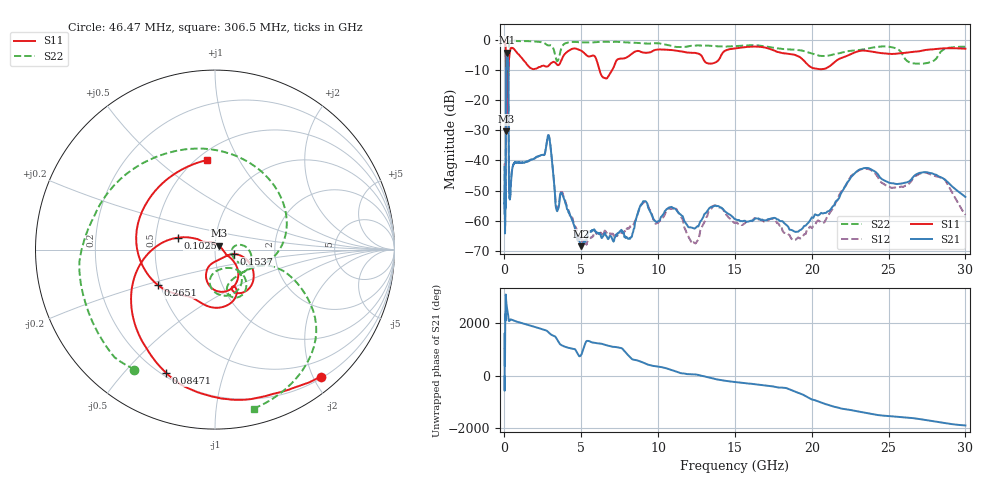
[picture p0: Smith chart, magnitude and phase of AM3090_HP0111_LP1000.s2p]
! Date/Time: Thu, Feb 28, 2019 2:01 PM
! Network Analyzer: Agilent Technologies E8364B Rev: A.07.50.67
! Sweep from 0.010 to 30.000 GHz, 1601 Points, Sweep Type: LOG
! Power Supply: 5.023 V, 0.002 A
# Hz S DB R 50
!freq MagS11 AngS11 MagS21 AngS21 MagS12 AngS12 MagS22 AngS22
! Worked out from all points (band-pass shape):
!   1601 points, 10 MHz to 30 GHz, reference 50 ohm
!   highest |S21| = -4.21 dB at 160.7 MHz (marker M1); lowest = -68.5 dB at 4.977 GHz (marker M2)
!   |S21| within 3 dB of the highest: 113.8 MHz to 240.5 MHz (126.7 MHz wide, 71.5 % of centre)
!   lowest |S11| = -30.3 dB at 110.4 MHz (marker M3), VSWR 1.06, Z = 52.1 + j2.32 ohm
!   |S11| at or under -10 dB: 100.6 MHz to 223.6 MHz (123 MHz wide, 75.9 % of centre); 234.8 MHz to 255.3 MHz (20.52 MHz wide, 8.37 % of centre); 6.184 GHz to 7.008 GHz (823.9 MHz wide, 12.5 % of centre)
!   |S22| runs from -20.7 to -0.1 dB; largest |S21 - S12| = 0.016
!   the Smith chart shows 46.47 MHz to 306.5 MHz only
!   S11 on the Smith chart (normalised r, x): 46.47 MHz: 0.22, -2.11; 84.71 MHz: 0.22, -0.66; 102.5 MHz: 0.65, +0.09; 153.7 MHz: 1.23, -0.06; 265.1 MHz: 0.48, -0.22; 306.5 MHz: 0.56, +0.75
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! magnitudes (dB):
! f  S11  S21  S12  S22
! 10 MHz  -0.3  -42.2  -41.0  -0.6
! 38.04 MHz  -0.5  -64.2  -59.5  -1.4
! 46.47 MHz  -0.7  -51.7  -51.5  -1.9
! 84.71 MHz  -2.6  -52.7  -51.1  -4.9
! 102.5 MHz  -13.3  -16.5  -16.4  -11.4
! 110.4 MHz  -30.3  -8.5  -8.5  -20.4
! 125.2 MHz  -12.5  -5.6  -5.6  -14.3
! 144.7 MHz  -24.1  -4.5  -4.4  -14.8
! 153.7 MHz  -19.4  -4.2  -4.2  -14.7
! 160.7 MHz  -13.9  -4.2  -4.2  -13.5
! 238.7 MHz  -10.3  -7.0  -7.0  -12.2
! 265.1 MHz  -8.5  -19.3  -19.2  -7.3
! 306.5 MHz  -6.0  -50.3  -50.7  -0.8
! 550.5 MHz  -2.7  -41.7  -41.8  -0.2
! 2.084 GHz  -9.5  -38.8  -38.9  -0.5
! 2.884 GHz  -8.5  -31.8  -31.7  -1.8
! 3.402 GHz  -8.0  -56.7  -55.7  -6.9
! 4.977 GHz  -3.5  -68.5  -66.0  -0.7
! 7.926 GHz  -5.8  -65.4  -63.1  -0.8
! 18.93 GHz  -5.0  -63.7  -66.4  -3.2
! 23.36 GHz  -3.5  -42.6  -42.8  -3.1
! 30 GHz  -2.9  -52.1  -58.1  -2.2
